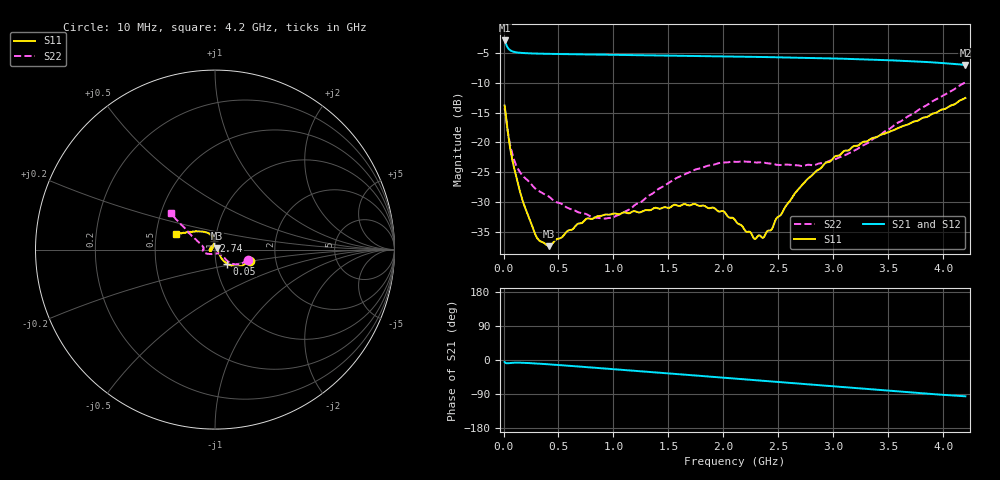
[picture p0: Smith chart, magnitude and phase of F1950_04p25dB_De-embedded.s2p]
! Integrated Device Technology
! Corporate Headquarters
! 6024 Silver Creek Valley Road
! San Jose, CA 95138  USA
! Phone:  1-408-284-8200
! Toll Free:  1-800-223-1366
! Webpage:  http://www.idt.com/
! Timing and RF Division
! 515 Groton Road, Suite 102
! Westford, MA 01886-6024
! Device:  F1950
! Description: 7-bit 0.25 dB Digital Step Attenuator
! Frequency:  150.0 -  4000.00 MHz
! Package:  4x4 mm Thin QFN Plastic Package: 24 pin
! Ports:  2 RF, 12 DC
!  Pin  1  = D0
!  Pin  2  = VDD
!  Pin  3  = Vmode
!  Pin  4  = GND
!  Pin  5  = RF1  =  Port 1
!  Pin  6  = GND
!  Pin  7  = GND
!  Pin  8  = GND
!  Pin  9  = GND
!  Pin 10  = GND
!  Pin 11  = GND
!  Pin 12  = GND
!  Pin 13  = GND
!  Pin 14  = RF2  =  Port 2
!  Pin 15  = GND
!  Pin 16  = LE
!  Pin 17  = CLK
!  Pin 18  = DATE
!  Pin 19  = D6
!  Pin 20  = D5
!  Pin 21  = D4
!  Pin 22  = D3
!  Pin 23  = D2
!  Pin 24  = D1
! State:  17
! Atten State:  4.25 dB
! Voltage:  +5.00 Volts
! Current:  Not Measured mA
! Data:  The device was measured on a the F195X evaluation board which has
!  individual transmission lines to the RF pins.  Data was collected
!  using a calibrated network analyzer.  The evaluation board was
!  de-embedded using a TRL calibration technique.
!  The reference plane is the edge of the package pin.
! Misc:  Board 2019
!  Action Tracker AT0250
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# GHz S dB R 50
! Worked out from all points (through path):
!   420 points, 10 MHz to 4.2 GHz, reference 50 ohm
!   highest |S21| = -2.84 dB at 10 MHz (marker M1); lowest = -7.0 dB at 4.2 GHz (marker M2)
!   group delay of S21, straight-line fit = 62.1 ps
!   lowest |S11| = -37.5 dB at 410 MHz (marker M3), VSWR 1.03, Z = 51.1 + j0.754 ohm
!   |S11| at or under -10 dB: start of sweep to end of sweep
!   |S22| runs from -32.8 to -9.9 dB; largest |S21 - S12| = 0.00067
!   S11 on the Smith chart (normalised r, x): 10 MHz: 1.47, -0.19; 50 MHz: 1.13, -0.18; 2.74 GHz: 0.98, +0.09; 4.2 GHz: 0.63, +0.12
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0.01  -13.79 -17.4  -2.84 -5.3  -2.84 -5.3  -14.26 -16.7
0.05  -19.72 -49.4  -4.33 -8.3  -4.33 -8.3  -19.41 -42.0
0.08  -22.96 -53.4  -4.68 -7.5  -4.67 -7.5  -21.95 -42.1
0.11  -25.30 -53.0  -4.82 -7.1  -4.82 -7.1  -23.65 -40.0
0.2  -31.17 -36.9  -4.98 -7.6  -4.98 -7.7  -26.06 -39.7
0.31  -36.22 -5.7  -5.06 -9.5  -5.06 -9.4  -28.07 -39.3
0.41  -37.47 33.4  -5.10 -11.4  -5.10 -11.4  -29.08 -39.6
0.71  -33.60 96.8  -5.18 -17.8  -5.18 -17.8  -31.89 -56.1
0.82  -32.77 107.2  -5.20 -20.2  -5.20 -20.2  -32.65 -67.8
0.99  -32.03 123.7  -5.25 -24.0  -5.25 -24.0  -32.66 -92.9
1.41  -31.13 169.1  -5.35 -33.3  -5.35 -33.3  -27.83 -143.3
1.74  -30.38 -168.4  -5.43 -40.8  -5.43 -40.8  -24.60 -160.7
2  -31.57 -165.3  -5.51 -46.7  -5.51 -46.7  -23.40 -169.0
2.11  -33.20 -168.0  -5.55 -49.2  -5.54 -49.2  -23.28 -171.8
2.28  -36.23 164.4  -5.60 -53.0  -5.60 -53.0  -23.37 -175.3
2.36  -36.07 143.6  -5.63 -54.8  -5.63 -54.9  -23.37 -177.1
2.44  -34.62 121.4  -5.65 -56.6  -5.65 -56.6  -23.58 -178.9
2.74  -26.66 97.5  -5.76 -63.5  -5.76 -63.6  -23.90 171.7
2.81  -25.46 97.1  -5.79 -65.1  -5.79 -65.2  -23.86 170.1
3.1  -21.42 105.5  -5.92 -71.9  -5.92 -71.9  -22.20 162.1
3.51  -18.17 125.2  -6.18 -81.3  -6.17 -81.4  -17.74 151.1
4.2  -12.52 158.0  -6.97 -95.7  -6.96 -95.8  -9.90 140.8
